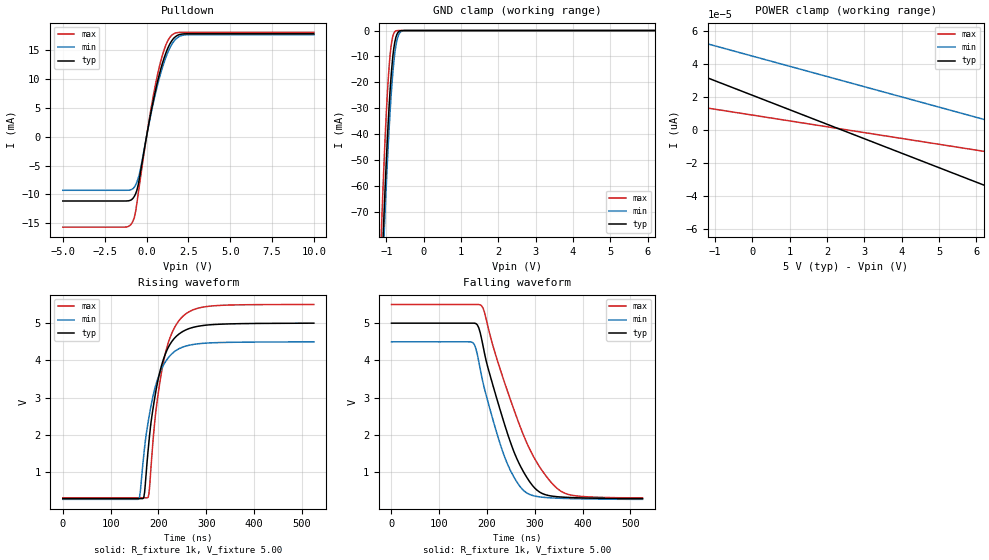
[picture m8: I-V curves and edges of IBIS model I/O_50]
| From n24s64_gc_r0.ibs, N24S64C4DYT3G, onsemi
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|//////////////////////////////////////////////////////////////////////////////
|//////////////////////////////////////////////////////////////////////////////
[Model] I/O_50
Model_type I/O_open_drain
Vinh = 3.50
Vinl = 1.50
Vmeas = 2.50
Vref = 5.00
Rref = 1000
Cref = 100pF
|  variable   typ   min   max
C_comp   8pF   8pF   8pF
|//////////////////////////////////////////////////////////////////////////////
[Temperature Range]   25   85   -40
|//////////////////////////////////////////////////////////////////////////////
[Voltage Range]   5.00V   4.50V   5.50V
|//////////////////////////////////////////////////////////////////////////////
[Pulldown Reference]   0V   0V   0V
|//////////////////////////////////////////////////////////////////////////////
[POWER Clamp Reference] 5.00V   4.50V   5.50V
|//////////////////////////////////////////////////////////////////////////////
[GND Clamp Reference]   0V   0V   0V
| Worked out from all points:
|   slope of the pulldown table from 0 to 0.75 V, typ, clamps not added: 70.7 ohm
|   GND clamp passes 1 mA (typ) near -0.70 V on its own axis
|   falling waveform, R_fixture 1k, V_fixture 5.00: 20-80 % time 70.2ns typ, 58.9ns min, 89.5ns max; typ from 5 V to 0.3 V
|   rising waveform, R_fixture 1k, V_fixture 5.00: 20-80 % time 35.2ns typ, 36ns min, 34.7ns max; typ from 0.3 V to 5 V
|//////////////////////////////////////////////////////////////////////////////
[Pulldown]
|   Voltage   I(typ)   I(min)   I(max)
-5V       -11.15mA   -9.288mA   -15.68mA
-1.25V    -11.14mA   -9.287mA   -15.66mA
-875mV    -10.87mA   -9.132mA   -14.99mA
-650mV    -9.896mA   -8.37mA    -12.96mA
-425mV    -7.274mA   -6.456mA   -8.43mA
175mV     2.813mA    2.624mA    3.208mA
625mV     9.136mA    8.56mA     10.31mA
1.075V    13.85mA    13.1mA     15.27mA
1.525V    16.7mA     16.08mA    17.64mA
1.9V      17.64mA    17.27mA    18.07mA
2.35V     17.84mA    17.66mA    18.1mA
10V       17.84mA    17.68mA    18.1mA
|//////////////////////////////////////////////////////////////////////////////
[GND Clamp]
|   Voltage   I(typ)   I(min)   I(max)
-5V       -1.529A    -1.535A    -1.509A
-1.15V    -102.2mA   -110.9mA   -83.75mA
-1.125V   -92.94mA   -101.6mA   -73.79mA
-1.075V   -74.71mA   -83.64mA   -55.14mA
-1.05V    -65.92mA   -75.11mA   -46.55mA
-975mV    -42.05mA   -51.26mA   -24.48mA
-925mV    -28.63mA   -37.32mA   -13.61mA
-825mV    -9.591mA   -15.86mA   -2.03mA
-750mV    -2.854mA   -6.231mA   -166uA
-650mV    -231uA     -1.049mA   -1.835uA
-500mV    -938.1nA   -12.88uA   -4.117nA
10V       64.9pA     78.81pA    24.87pA
|//////////////////////////////////////////////////////////////////////////////
[POWER Clamp]
|   Voltage   I(typ)   I(min)   I(max)
-5V       53.88nA    58.4nA     40.05nA
-2.975V   63.47pA    63.16pA    230.5pA
-2.95V    60.47pA    63pA       204.4pA
-2.875V   52.61pA    62.54pA    144.1pA
-2.825V   48.91pA    62.23pA    112.7pA
-2.775V   46.59pA    61.92pA    89.05pA
-2.7V     44.88pA    61.45pA    65.64pA
-2.525V   43.13pA    60.37pA    34.19pA
-2.375V   41.81pA    59.44pA    19.47pA
-2.15V    39.84pA    58.05pA    16.53pA
5.225V    -25.01pA   12.35pA    -9.626pA
10V       -67pA      -17.24pA   -26.56pA
|//////////////////////////////////////////////////////////////////////////////
|//////////////////////////////////////////////////////////////////////////////
[Ramp]
|  variable   typ   min   max
dV/dt_r   2.820E+00/3.450E-08  2.532E+00/3.600E-08  3.108E+00/3.450E-08
dV/dt_f   2.820E+00/7.200E-08  2.532E+00/6.000E-08  3.108E+00/9.000E-08
R_load = 1k
|//////////////////////////////////////////////////////////////////////////////
|//////////////////////////////////////////////////////////////////////////////
[Falling Waveform]
R_fixture = 1k
V_fixture = 5.00
V_fixture_min = 4.50
V_fixture_max = 5.50
C_fixture = 0p
|   time   V(typ)   V(min)   V(max)
0s        5V         4.5V       5.5V
168ns     5V         4.492V     5.5V
177ns     4.987V     4.304V     5.5V
189ns     4.556V     3.557V     5.461V
201ns     3.848V     2.934V     4.953V
243ns     2.036V     1.22V      3.171V
273ns     1.094V     564.4mV    2.107V
300ns     580.9mV    368.1mV    1.363V
366ns     333.3mV    302.6mV    428.7mV
525.5ns   300mV      280mV      320mV
|//////////////////////////////////////////////////////////////////////////////
[Rising Waveform]
R_fixture = 1k
V_fixture = 5.00
V_fixture_min = 4.50
V_fixture_max = 5.50
C_fixture = 0p
|   time   V(typ)   V(min)   V(max)
0s        300mV      280mV      320mV
159ns     300mV      290.1mV    320mV
169.5ns   344.6mV    1.495V     320mV
178.5ns   1.613V     2.355V     338.8mV
193.5ns   3.099V     3.299V     2.518V
210ns     4.015V     3.865V     3.932V
228ns     4.509V     4.178V     4.732V
255ns     4.806V     4.377V     5.228V
317ns     4.964V     4.476V     5.467V
525ns     5V         4.5V       5.5V
